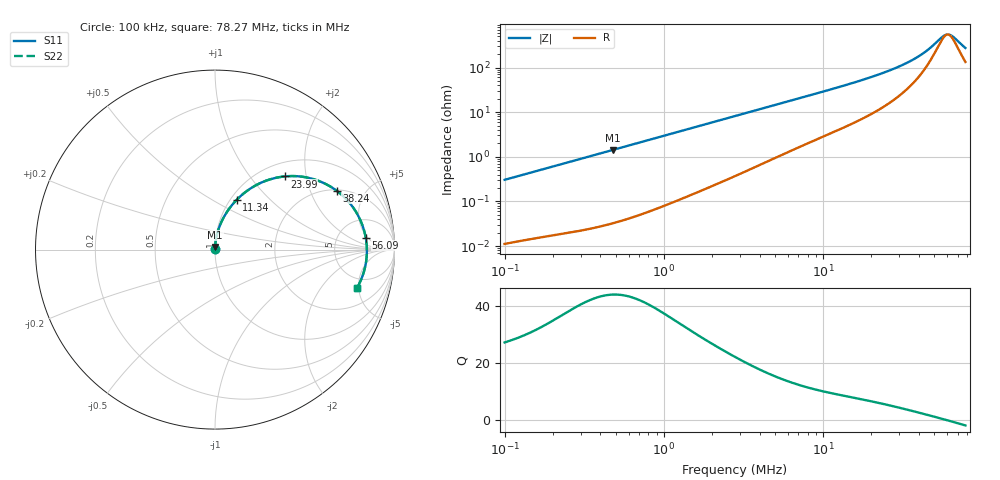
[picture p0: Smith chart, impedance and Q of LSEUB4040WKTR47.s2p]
! LSEUB4040WKTR47  S-PARAMETER MODEL  ( Standard Model )
! Model Generated by TAIYO YUDEN Corporation (http://www.ty-top.com)
! Version 1.0
! TAIYO YUDEN Control No. 20230502
! Copyright(c) 2023 TAIYO YUDEN CO.,LTD. All Rights Reserved.
! Product Description (link to TY-COMPAS)
! https://ds.yuden.co.jp/TYCOMPAS/or/detail?pn=LSEUB4040WKTR47M&u=M
! Products Name : Inductors
! Characteristics :
!  Inductance : 0.47 [uH] , SRF(min) : - [Hz] , DC Resistance(max) : 0.0065 [Ohm]
!  Rated Current : Saturation  14000 [mA] , Temp Rise  9900 [mA] (40 [degC])
!  Case Size : 4.0 x 4.0 / 0.157 x 0.157 [mm/inch] , Thickness : 2.0 / 0.079 [mm/inch]
!  (Conditions: Temperature = 25 [degC] , DC Bias Current = 0 [A])
! External Node Assignments :
!  1  o---GGG---o  2
! GND o---------o GND
! Frequency Range : 0.1MHz  -  78.268192MHz  [ 402 STEP ]
# MHz S RI R 50
! Freq[MHz].  S11 Real  S11 Imag  S21 Real  S21 Imag  S12 Real  S12 Imag  S22 Real  S22 Imag
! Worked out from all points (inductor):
!   401 points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, 100 kHz to 78.27 MHz, reference 50 ohm
!   read as one part in series: L = 482 nH near 103.4 kHz
!   highest Q = 44.1 at 478.6 kHz (marker M1), where L = 474 nH
!   self-resonance near 60.53 MHz
!   S11 on the Smith chart (normalised r, x): 100 kHz: 1.00, +0.01; 11.34 MHz: 1.07, +0.65; 23.99 MHz: 1.26, +1.51; 38.24 MHz: 2.04, +3.10; 56.09 MHz: 10, +4; 78.27 MHz: 3.67, -4.79
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0.1  0.000121 0.00304  0.9999 -0.00304  0.9999 -0.00304  0.000121 0.00304
0.305264  0.000307 0.00912  0.9997 -0.00912  0.9997 -0.00912  0.000307 0.00912
0.478622  0.000527 0.0143  0.9995 -0.0143  0.9995 -0.0143  0.000527 0.0143
0.931861  0.00148 0.0276  0.9985 -0.0276  0.9985 -0.0276  0.00148 0.0276
2.844635  0.0106 0.0821  0.9894 -0.0821  0.9894 -0.0821  0.0106 0.0821
5.011657  0.0295 0.1397  0.9705 -0.1397  0.9705 -0.1397  0.0295 0.1397
8.540203  0.075 0.2221  0.925 -0.2221  0.925 -0.2221  0.075 0.2221
11.33563  0.1206 0.2772  0.8794 -0.2772  0.8794 -0.2772  0.1206 0.2772
16.90677  0.2296 0.3594  0.7704 -0.3594  0.7704 -0.3594  0.2296 0.3594
20.30646  0.3043 0.3907  0.6957 -0.3907  0.6957 -0.3907  0.3043 0.3907
23.98689  0.388 0.4077  0.612 -0.4077  0.612 -0.4077  0.388 0.4077
26.07016  0.4353 0.4098  0.5647 -0.4098  0.5647 -0.4098  0.4353 0.4098
31.8384  0.5599 0.3891  0.4401 -0.3891  0.4401 -0.3891  0.5599 0.3891
38.24062  0.677 0.3288  0.323 -0.3288  0.323 -0.3288  0.677 0.3288
42.25992  0.7352 0.2768  0.2648 -0.2768  0.2648 -0.2768  0.7352 0.2768
45.93021  0.7772 0.2236  0.2228 -0.2236  0.2228 -0.2236  0.7772 0.2236
56.09266  0.84 0.0663  0.16 -0.0663  0.16 -0.0663  0.84 0.0663
59.95728  0.8461 0.00834  0.1539 -0.00834  0.1539 -0.00834  0.8461 0.00834
63.02949  0.8454 -0.0355  0.1546 0.0355  0.1546 0.0355  0.8454 -0.0355
66.25912  0.84 -0.079  0.16 0.079  0.16 0.079  0.84 -0.079
75.70375  0.8044 -0.1889  0.1956 0.1889  0.1956 0.1889  0.8044 -0.1889
78.26819  0.7911 -0.2141  0.2089 0.2141  0.2089 0.2141  0.7911 -0.2141
